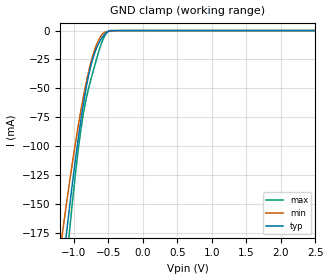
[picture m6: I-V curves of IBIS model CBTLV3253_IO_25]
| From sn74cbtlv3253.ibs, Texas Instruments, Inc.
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[Model]   CBTLV3253_IO_25
Model_type  Terminator
| variable   typ   min   max
C_comp   20.5pF   NA   NA
| C_tri-state   14.27pF   12.07pF   15.65pF
[Temperature Range]   40   100   -40
| Ambient temperature   25   85   -40
[Voltage range]   2.5   2.3   2.7
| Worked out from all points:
|   GND clamp passes 1 mA (typ) near -0.51 V on its own axis
[GND Clamp]
| CBTLV3253_IO_25
|   Voltage   I(typ)   I(min)   I(max)
-2.5V     -1.078A    -894mA     -1.299A
-1.18V    -214.3mA   -181.4mA   -248.8mA
-1.16V    -203.4mA   -172.5mA   -235.4mA
-1.1V     -171.5mA   -146.5mA   -196.3mA
-1.08V    -161.1mA   -138mA     -183.7mA
-1.06V    -151mA     -129.8mA   -171.3mA
-910mV    -81.74mA   -72.8mA    -90.44mA
-805mV    -43.94mA   -40.27mA   -54.38mA
-700mV    -19.43mA   -16.68mA   -30.58mA
-565mV    -3.933mA   -1.868mA   -5.854mA
-470mV    -91.79uA   -501.9uA   -30.24uA
2.5V      1.475nA    64.06nA    39.46pA
